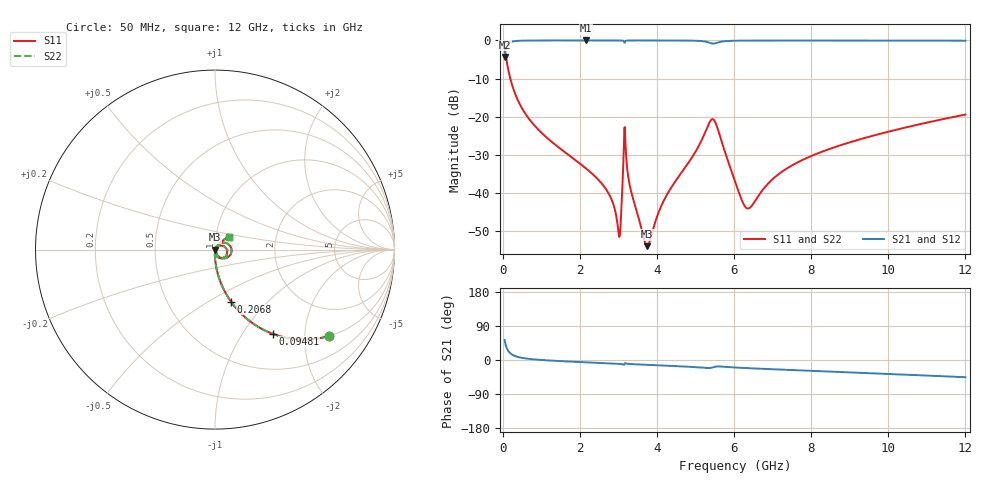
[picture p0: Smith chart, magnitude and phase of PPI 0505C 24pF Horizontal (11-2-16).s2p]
# MHz S MA R 50
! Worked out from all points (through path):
!   1601 points, 50 MHz to 12 GHz, reference 50 ohm
!   highest |S21| = -0.02 dB at 2.149 GHz (marker M1); lowest = -4.4 dB at 50 MHz (marker M2)
!   group delay of S21, straight-line fit = 11.9 ps
!   lowest |S11| = -54.0 dB at 3.747 GHz (marker M3), VSWR 1.00, Z = 50.2 - j0.0522 ohm
!   |S11| at or under -10 dB: 197.4 MHz to end of sweep
!   |S22| runs from -54.0 to -2.0 dB; largest |S21 - S12| = 0
!   S11 on the Smith chart (normalised r, x): 50 MHz: 0.99, -2.63; 94.81 MHz: 0.99, -1.39; 206.8 MHz: 0.99, -0.63; 12 GHz: 1.16, +0.17
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50  0.7969 -37.3  0.6039 52.7  0.6039 52.7  0.7969 -37.3
94.8125  0.5709 -55.5  0.8207 34.5  0.8207 34.5  0.5709 -55.5
206.8438  0.3031 -73.0  0.9525 16.9  0.9525 16.9  0.3031 -73.0
759.5312  0.08355 -87.2  0.9956 2.2  0.9956 2.2  0.08355 -87.2
2044.156  0.02333 -92.4  0.9983 -5.6  0.9983 -5.6  0.02333 -92.4
2148.719  0.02116 -92.4  0.9983 -6.1  0.9983 -6.1  0.02116 -92.4
2746.219  0.009854 -89.1  0.9981 -8.8  0.9981 -8.8  0.009854 -89.1
3007.625  0.00294 -46.2  0.9974 -10.2  0.9974 -10.2  0.00294 -46.2
3059.906  0.004026 25.7  0.9966 -10.6  0.9966 -10.6  0.004026 25.7
3142.062  0.03993 33.1  0.9714 -12.3  0.9714 -12.3  0.03993 33.1
3186.875  0.04144 -73.8  0.9816 -8.7  0.9816 -8.7  0.04144 -73.8
3328.781  0.01055 -89.2  0.9976 -10.7  0.9976 -10.7  0.01055 -89.2
3747.031  0.001999 -15.1  0.9978 -12.7  0.9978 -12.7  0.001999 -15.1
4038.312  0.005462 51.5  0.9975 -14.0  0.9975 -14.0  0.005462 51.5
5427.5  0.09231 -1.0  0.912 -20.1  0.912 -20.1  0.09231 -1.0
5547  0.07675 -38.1  0.9276 -17.2  0.9276 -17.2  0.07675 -38.1
6025  0.01418 -63.8  0.9894 -19.8  0.9894 -19.8  0.01418 -63.8
6383.5  0.006264 -2.0  0.9937 -21.6  0.9937 -21.6  0.006264 -2.0
7085.562  0.01649 51.3  0.9954 -24.7  0.9954 -24.7  0.01649 51.3
8019.156  0.03069 54.9  0.9955 -28.6  0.9955 -28.6  0.03069 54.9
10013.31  0.06366 49.9  0.9938 -36.8  0.9938 -36.8  0.06366 49.9
12000  0.1066 42.3  0.9895 -45.5  0.9895 -45.5  0.1066 42.3
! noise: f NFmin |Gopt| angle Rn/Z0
50  0.0003847  0.8642  0.9861  0.0006077
1372  0.00393  0.6703  4.887  0.002288
2701  0.006749  0.6318  9.278  0.003422
4031  0.009698  0.6219  13.67  0.004725
5360  0.05962  0.9046  18.13  0.1336
6682  0.01777  0.656  22.46  0.00949
8012  0.01692  0.5885  26.58  0.007147
9341  0.01829  0.5672  30.59  0.007133
1.067e+04  0.02013  0.5589  34.49  0.00753
1.2e+04  0.02221  0.5571  38.26  0.008102
